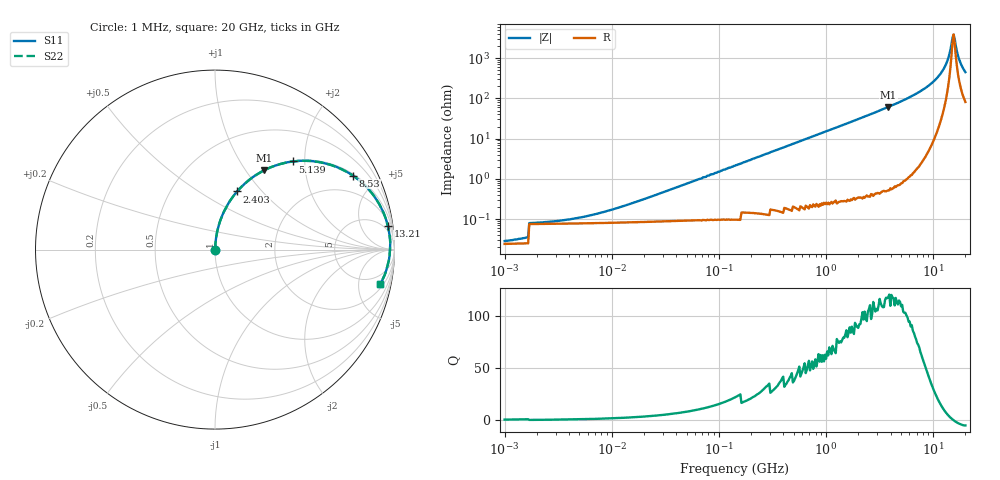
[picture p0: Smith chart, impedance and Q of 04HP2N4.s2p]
# MHz S MA R 50
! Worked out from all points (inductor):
!   431 points, 1 MHz to 20 GHz, reference 50 ohm
!   read as one part in series: L = 2.4 nH near 16.99 MHz
!   highest Q = 118 at 3.809 GHz (marker M1), where L = 2.56 nH
!   self-resonance near 15.17 GHz
!   S11 on the Smith chart (normalised r, x): 1 MHz: 1.00, +0.00; 2.403 GHz: 1.01, +0.74; 5.139 GHz: 1.02, +1.74; 8.53 GHz: 1.07, +3.69; 13.21 GHz: 3, +14; 20 GHz: 2.62, -8.86
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1  0.0005048 17.4  1 -0.0  1 -0.0  0.0005048 17.4
2.345  0.0006243 34.5  0.999 -0.0  0.999 -0.0  0.0006243 34.5
5.25  0.0009704 54.6  0.999 -0.0  0.999 -0.0  0.0009704 54.6
27.564  0.00422 79.6  0.999 -0.2  0.999 -0.2  0.00422 79.6
144.716  0.022 85.7  0.999 -1.2  0.999 -1.2  0.022 85.7
742.485  0.111 82.5  0.992 -6.4  0.992 -6.4  0.111 82.5
1481.697  0.219 76.6  0.973 -12.7  0.973 -12.7  0.219 76.6
2403.309  0.347 69.1  0.934 -20.3  0.934 -20.3  0.347 69.1
3809.408  0.52 58.2  0.85 -31.3  0.85 -31.3  0.52 58.2
3898.162  0.53 57.5  0.844 -32.0  0.844 -32.0  0.53 57.5
5139.119  0.654 48.6  0.751 -40.8  0.751 -40.8  0.654 48.6
6620.869  0.769 39.0  0.63 -50.3  0.63 -50.3  0.769 39.0
8529.849  0.872 28.2  0.473 -60.7  0.473 -60.7  0.872 28.2
11245.28  0.95 15.4  0.266 -71.6  0.266 -71.6  0.95 15.4
13212.56  0.972 7.7  0.135 -74.4  0.135 -74.4  0.972 7.7
13835.4  0.975 5.5  0.097 -72.6  0.097 -72.6  0.975 5.5
14825.14  0.977 2.2  0.044 -56.7  0.044 -56.7  0.977 2.2
15524  0.975 -0.0  0.025 1.5  0.025 1.5  0.975 -0.0
15885.69  0.974 -1.1  0.032 36.5  0.032 36.5  0.974 -1.1
17824.53  0.962 -6.6  0.118 68.1  0.118 68.1  0.962 -6.6
19099.64  0.95 -9.8  0.173 68.5  0.173 68.5  0.95 -9.8
20000  0.941 -11.9  0.209 67.6  0.209 67.6  0.941 -11.9
